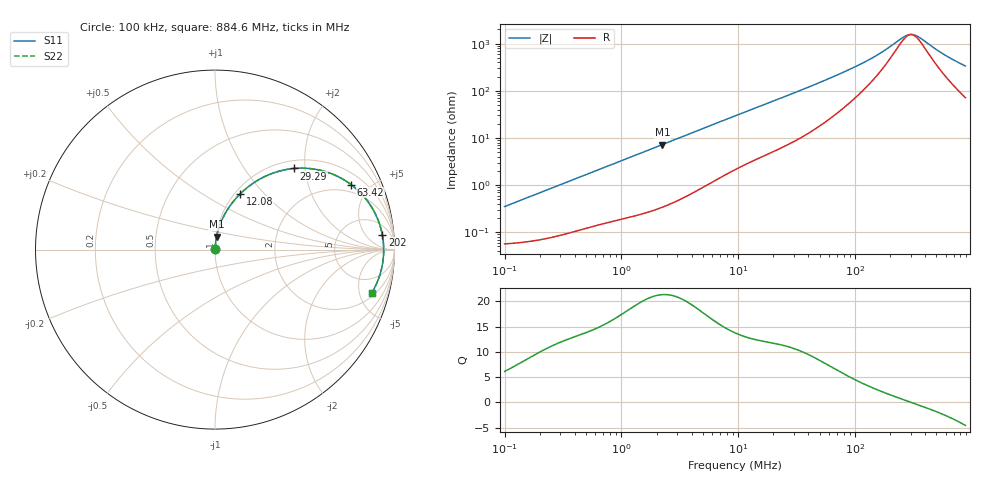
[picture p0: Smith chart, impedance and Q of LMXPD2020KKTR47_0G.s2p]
! LMXPD2020KKTR47_0G  S-PARAMETER MODEL  ( General Type )
! Model Generated by TAIYO YUDEN Corporation (https://www.yuden.co.jp/en/)
! Version 1.0
! TAIYO YUDEN Control No. 191023NI43SB-FBB
! Copyright(c) 2019 TAIYO YUDEN CO.,LTD. All Rights Reserved.
! Product Description (link to TY-COMPAS)
! https://ds.yuden.co.jp/TYCOMPAS/or/detail?pn=LMXPD2020KKTR47N0G&u=M
! Products Name : Inductors
! Characteristics :
!  Inductance : 0.47 uH , SRF(min) : -Hz , DC Resistance(max) : 0.0624 Ohm
!  Rated Current : Saturation :2100 mA , Temp Rise : 2000 mA (40 degC)
!  Case Size : 2.0 x 2.0 / 0.079 x 0.079 [mm/inch] , Thickness : 1 / 0.039 [mm/inch]
!  (Conditions: Temperature = 25 degC , DC Bias Current/Voltage = 0A / 0V)
! External Node Assignments :
!  1  o---GGG---o  2
! GND o---------o GND
! Frequency Range : 0.1MHz  -  884.637303MHz  [ 402 STEP ]
# MHz S RI R 50
! Freq[MHz].  S11 Real  S11 Imag  S21 Real  S21 Imag  S12 Real  S12 Imag  S22 Real  S22 Imag
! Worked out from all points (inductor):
!   401 points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, 100 kHz to 884.6 MHz, reference 50 ohm
!   read as one part in series: L = 551 nH near 104.6 kHz
!   highest Q = 21.3 at 2.248 MHz (marker M1), where L = 514 nH
!   self-resonance near 302.8 MHz
!   S11 on the Smith chart (normalised r, x): 100 kHz: 1.00, +0.01; 12.08 MHz: 1.06, +0.74; 29.29 MHz: 1.16, +1.74; 63.42 MHz: 1.55, +3.82; 202 MHz: 11, +14; 884.6 MHz: 2.43, -6.56
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0.1  0.000578 0.00346  0.9994 -0.00346  0.9994 -0.00346  0.000578 0.00346
0.45823  0.00138 0.0154  0.9986 -0.0154  0.9986 -0.0154  0.00138 0.0154
2.099744  0.00773 0.0671  0.9923 -0.0671  0.9923 -0.0671  0.00773 0.0671
2.247849  0.00858 0.0717  0.9914 -0.0717  0.9914 -0.0717  0.00858 0.0717
4.650593  0.029 0.1427  0.971 -0.1427  0.971 -0.1427  0.029 0.1427
9.405516  0.0948 0.2588  0.9052 -0.2588  0.9052 -0.2588  0.0948 0.2588
12.07588  0.1395 0.3096  0.8605 -0.3096  0.8605 -0.3096  0.1395 0.3096
18.59474  0.2569 0.3968  0.7431 -0.3968  0.7431 -0.3968  0.2569 0.3968
29.2906  0.4389 0.4519  0.5611 -0.4519  0.5611 -0.4519  0.4389 0.4519
43.09886  0.6123 0.4353  0.3877 -0.4353  0.3877 -0.4353  0.6123 0.4353
63.41665  0.7579 0.3625  0.2421 -0.3625  0.2421 -0.3625  0.7579 0.3625
85.20659  0.8358 0.2882  0.1642 -0.2882  0.1642 -0.2882  0.8358 0.2882
119.8055  0.8924 0.2012  0.1076 -0.2012  0.1076 -0.2012  0.8924 0.2012
157.3547  0.9185 0.1367  0.0815 -0.1367  0.0815 -0.1367  0.9185 0.1367
197.4918  0.9312 0.087  0.0688 -0.087  0.0688 -0.087  0.9312 0.087
202.03  0.9322 0.0822  0.0678 -0.0822  0.0678 -0.0822  0.9322 0.0822
271.4475  0.9393 0.0218  0.0607 -0.0218  0.0607 -0.0218  0.9393 0.0218
297.2716  0.9399 0.00367  0.0601 -0.00367  0.0601 -0.00367  0.9399 0.00367
318.2396  0.9399 -0.00992  0.0601 0.00992  0.0601 0.00992  0.9399 -0.00992
356.524  0.9389 -0.0327  0.0611 0.0327  0.0611 0.0327  0.9389 -0.0327
601.2121  0.9175 -0.1443  0.0825 0.1443  0.0825 0.1443  0.9175 -0.1443
884.6373  0.8747 -0.2395  0.1253 0.2395  0.1253 0.2395  0.8747 -0.2395
